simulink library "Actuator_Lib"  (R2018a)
settings: Solver=VariableStepAuto  StartTime=0.0  StopTime=10.0  RelTol=1e-3

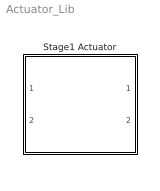
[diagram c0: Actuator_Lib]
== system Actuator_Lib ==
  Stage1 Actuator : Subsystem

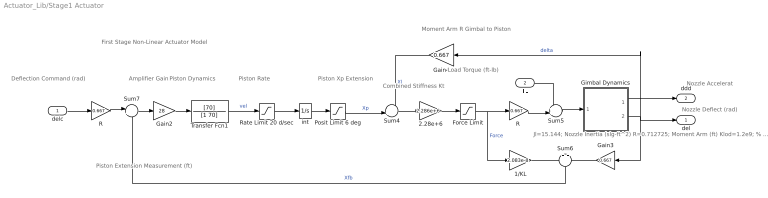
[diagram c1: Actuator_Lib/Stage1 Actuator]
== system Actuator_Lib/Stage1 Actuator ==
  note: Piston Extension Measurement (ft)
  note: Moment Arm R Gimbal to Piston
  note: Load Torque (ft-lb)
  note: Amplifier Gain
  note: Piston Xp Extension
  note: First Stage Non-Linear Actuator Model
  note: Piston Dynamics
  note: Piston Rate
  note: Deflection Command (rad)
  note: Nozzle Accelerat
  note: Nozzle Deflect (rad)
  note: Combined Stiffness Kt
  note: Jl=15.144; Nozzle Inertia (slg-ft^2) R=0.712725; Moment Arm (ft) Klod=1.2e9; % Load Stiffness Kact=2.4e6; % Piston Stiffness Kbck=1.122e6; % Backup Structure Stiffn Kti=(1/Klod)+(1/Kact)+(1/Kbck); Kt=1/Kti; % Combined Structural Stiffness Ka=26; % Amplifier Gain
  delc : Inport
  TL : Inport  Port=2
  1/KL : Gain  Gain=2.083e-8
  2.28e+6 : Gain  Gain=2.286e+6
  Force Limit : Saturate  UpperLimit=4000  LowerLimit=-4000
  Gain2 : Gain  Gain=28
  Gain3 : Gain  Gain=0.667
  Gain4 : Gain  Gain=0.667
  Gimbal Dynamics : Subsystem
  Posit Limit 6 deg : Saturate  UpperLimit=0.075  LowerLimit=-0.075
  R : Gain  Gain=0.667
  "R " : Gain  Gain=0.667
  Rate Limit 20 d/sec : Saturate  UpperLimit=0.23  LowerLimit=-0.23
  Sum4 : Sum  Inputs=-+|
  Sum5 : Sum  Inputs=++|
  Sum6 : Sum  Inputs=+|+
  Sum7 : Sum  Inputs=|+-
  Transfer Fcn1 : TransferFcn  Numerator=[70]  Denominator=[1 70]
  int : Integrator
  del : Outport
  ddd : Outport  Port=2
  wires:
  Gimbal Dynamics/2(" delta") -> Gain3/1, del/1, Gain4/1  "delta"
  Transfer Fcn1/1 -> Rate Limit 20 d/sec/1  "vel"
  Sum5/1 -> Gimbal Dynamics/1(Tin)
  Gimbal Dynamics/1(Axel) -> ddd/1
  R/1 -> Sum7/1
  Sum4/1 -> 2.28e+6/1
  Gain2/1 -> Transfer Fcn1/1
  Sum7/1 -> Gain2/1
  TL/1 -> Sum5/1
  Gain3/1 -> Sum6/2
  Gain4/1 -> Sum4/1  "Xl"
  1/KL/1 -> Sum6/1
  2.28e+6/1 -> Force Limit/1
  Force Limit/1 -> 1/KL/1, "R "/1  "Force"
  int/1 -> Posit Limit 6 deg/1
  Sum6/1 -> Sum7/2  "Xfb"
  Rate Limit 20 d/sec/1 -> int/1
  Posit Limit 6 deg/1 -> Sum4/2  "Xp"
  delc/1 -> R/1
  "R "/1 -> Sum5/2

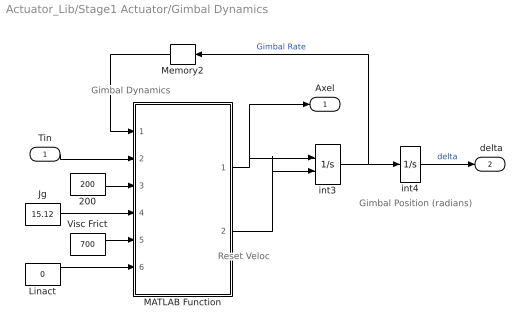
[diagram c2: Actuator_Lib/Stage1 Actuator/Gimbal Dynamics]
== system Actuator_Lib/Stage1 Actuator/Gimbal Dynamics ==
  note: Gimbal Dynamics
  note: Gimbal Position (radians)
  note: Reset Veloc
  Tin : Inport
  200 : Constant  Value=200
  Jg : Constant  Value=15.12
  Linact : Constant  Value=0
  MATLAB Function : MATLAB Function  TreatAsAtomicUnit=on
  Memory2 : Memory
  Visc Frict : Constant  Value=700
  int3 : Integrator  ExternalReset=rising
  int4 : Integrator
  Axel : Outport
  " delta" : Outport  Port=2
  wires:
  Memory2/1 -> MATLAB Function/1(Rate)
  Jg/1 -> MATLAB Function/4(Jg)
  MATLAB Function/1(Axel) -> Axel/1, int3/1
  Tin/1 -> MATLAB Function/2(Tin)
  int3/1 -> Memory2/1, int4/1  "Gimbal Rate"
  int4/1 -> " delta"/1  "delta"
  MATLAB Function/2(Rvel) -> int3/2
  Linact/1 -> MATLAB Function/6(Lin)
  200/1 -> MATLAB Function/3(Tst)
  Visc Frict/1 -> MATLAB Function/5(Bvf)

== matlab function Actuator_Lib/Stage1 Actuator/Gimbal 
Dynamics/MATLAB Function ==
function [Axel,Rvel] = Gimbal(Rate,Tin,Tst,Jg,Bvf,Lin)    
% Gimbal Friction Dynamics
% Tin:  Input Torque (ft-lb)
% Rate: Gimbal Rate (rad/sec)
% Bvf:  Viscous Friction
% Tfr:  Gimbal Friction Torque (ft-lb)
% axel: Gimbal Acceleration (ft/sec2)
% Tst:  Gimbal Static Friction Torq (ft-lb)
% Jg:   Gimbal Inertia (slg-ft^2)

if Lin>0.5                                % Linear Actuator (1)
    Tfr=Bvf*Rate;                         % Viscous Friction Torque
    Axel=(Tin-Tfr)/Jg;                    % Gimbal Acceleration
    Rvel=0;                               % Dont Reset
else                                      % Non-Linear Actuator (0)
    if abs(Rate)<0.01                     % If Not Moving Much
        if abs(Tin)>Tst*1.05              % Exceeds Stiction, Start Moving
            Tfr=Tst*sign(Tin);            % Friction Torque resist motion
            Axel=(Tin-Tfr)/Jg;            % Gimbal Acceleration
            Rvel=0;
        else                              % Stop the Motion
            Axel=0;
            Tfr=0;                        % No Frict when not moving
            Rvel=1;                       % Reset Velocity to Zero
        end
        
    else                                  % Gimbal is Fast Enough
        Tfr=Tst*sign(Rate);               % Friction Torque resist motion
        Axel=(Tin-Tfr)/Jg;                % Gimbal Acceleration
        Rvel=0;
    end
end
end
